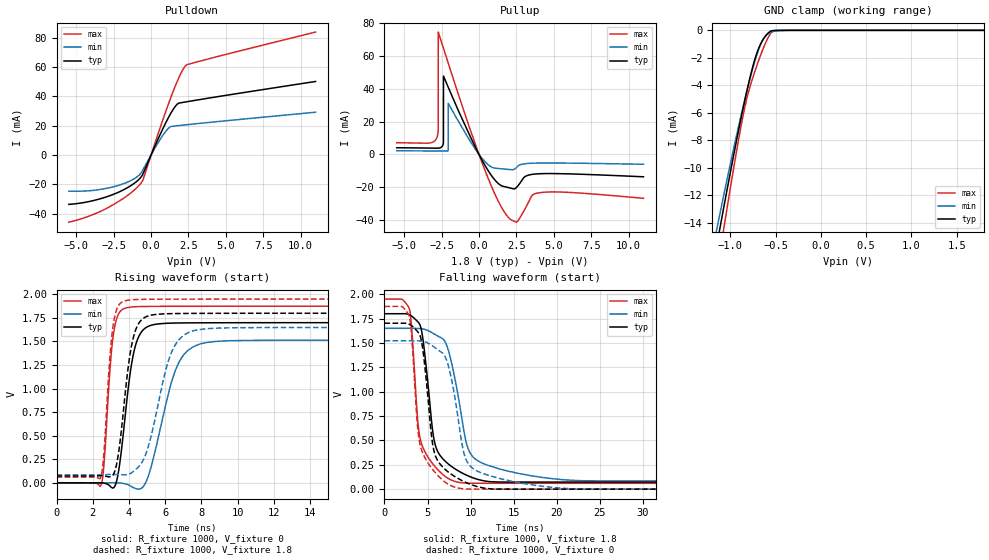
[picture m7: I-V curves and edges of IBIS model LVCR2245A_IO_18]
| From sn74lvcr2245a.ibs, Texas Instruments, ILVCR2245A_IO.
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[Model]   LVCR2245A_IO_18
Model_type  I/O
Vinl=0.5775
Vinh=1.2675
Enable   Active-Low
Vref =   0
Rref =   1000
Cref =   30p
Vmeas =   0.9
| variable   typ   min   max
C_comp   5.81pF   5.64pF   6.29pF
| C_pullup   5.68pF   4.72pF   6.93pF
| C_pulldown   4.75pF   4.06pF   6.38pF
| C_tri-state   5.81pF   5.64pF   6.29pF
[Temperature Range]   40   100   -40
| Ambient temperature   25   85   -40
[Voltage range]   1.8   1.65   1.95
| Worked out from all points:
|   slope of the pulldown table from 0 to 0.27 V, typ, clamps not added: 42.5 ohm
|   slope of the pullup table from 0 to 0.27 V, typ, clamps not added: 58.8 ohm
|   GND clamp passes 1 mA (typ) near -0.67 V on its own axis
|   rising waveform, R_fixture 1000, V_fixture 0: 20-80 % time 659ps typ, 1.2ns min, 405ps max; typ from 0 V to 1.7 V
|   falling waveform, R_fixture 1000, V_fixture 1.8: 20-80 % time 1.44ns typ, 2.12ns min, 1.2ns max; typ from 1.8 V to 0.073 V
|   rising waveform, R_fixture 1000, V_fixture 1.8: 20-80 % time 647ps typ, 1.17ns min, 400ps max; typ from 0.073 V to 1.8 V
|   falling waveform, R_fixture 1000, V_fixture 0: 20-80 % time 1.37ns typ, 1.91ns min, 1.21ns max; typ from 1.7 V to 0 V
[GND Clamp]
| LVCR2245A_IO_18
|   Voltage   I(typ)   I(min)   I(max)
-5.5V     -191mA     -172.6mA   -219.2mA
-1.155V   -15.81mA   -14.6mA    -17.82mA
-1.115V   -14.36mA   -13.31mA   -16.15mA
-1.08V    -13.11mA   -12.19mA   -14.7mA
-1.045V   -11.88mA   -11.09mA   -13.26mA
-935mV    -8.103mA   -7.723mA   -8.901mA
-855mV    -5.522mA   -5.416mA   -6.041mA
-810mV    -4.171mA   -4.195mA   -4.729mA
-745mV    -2.448mA   -2.581mA   -3.287mA
-640mV    -679.9uA   -662.4uA   -1.354mA
-530mV    -22.6uA    -93.97uA   -52.84uA
1.8V      36.78pA    10.02nA    -1.384nA
[Pulldown]
| LVCR2245A_IO_18
|   Voltage   I(typ)   I(min)   I(max)
-5.5V     -33.74mA   -24.8mA    -45.91mA
-3.97V    -31.41mA   -24.29mA   -41.06mA
-2.605V   -27.23mA   -21.94mA   -34.38mA
-1.375V   -21.08mA   -17.61mA   -26.1mA
-670mV    -15.02mA   -12.24mA   -19.16mA
-520mV    -12.37mA   -9.63mA    -16.31mA
495mV     11.51mA    8.797mA    15.32mA
1.11V     24.56mA    17.67mA    33.39mA
1.745V    34.65mA    19.96mA    50.16mA
2.1V      35.85mA    20.36mA    57.82mA
2.355V    36.3mA     20.63mA    61.42mA
11V       50.2mA     29.22mA    83.93mA
[Pullup]
| LVCR2245A_IO_18
|   Voltage   I(typ)   I(min)   I(max)
-5.5V     4.122mA    2.276mA    7.196mA
-2.81V    3.859mA    2.118mA    10.5mA
-2.73V    3.868mA    2.112mA    14.82mA
-2.725V   3.87mA     2.111mA    74.73mA
-2.385V   7.027mA    2.085mA    65.04mA
-2.38V    7.733mA    2.085mA    64.9mA
-2.375V   47.86mA    2.084mA    64.76mA
-2.06V    41.1mA     2.782mA    55.79mA
-2.055V   40.99mA    31.29mA    55.65mA
2.09V     -20.49mA   -9.224mA   -39.54mA
4.04V     -11.77mA   -5.224mA   -23.37mA
11V       -13.62mA   -5.978mA   -26.77mA
[Ramp]
| LVCR2245A_IO_18
| variable   typ   min   max
dV/dt_r   1.05/6.80E-10   0.95/1.24E-09   1.15/4.18E-10
dV/dt_f   1.04/1.44E-09   0.94/2.12E-09   1.13/1.20E-09
R_load = 1000
[Rising Waveform]
| LVCR2245A_IO_18
R_fixture =   1000
C_fixture =   0
L_fixture =   0
V_fixture =   0
V_fixture_min = 0
V_fixture_max = 0
|   Time   V(typ)   V(min)   V(max)
0s        702pV      3.493nV    28.21nV
2.46ns    -115.1uV   -529uV     -22.19mV
3.155ns   -51.34mV   393.3uV    1.591V
3.465ns   169.6mV    -1.365mV   1.805V
3.915ns   929.8mV    -16.65mV   1.859V
4.32ns    1.427V     -56.76mV   1.868V
4.83ns    1.631V     -29.83mV   1.871V
6.655ns   1.696V     1.235V     1.873V
8.27ns    1.698V     1.488V     1.874V
50ns      1.7V       1.515V     1.874V
[Falling Waveform]
| LVCR2245A_IO_18
R_fixture =   1000
C_fixture =   0
L_fixture =   0
V_fixture =   1.8
V_fixture_min = 1.65
V_fixture_max = 1.95
|   Time   V(typ)   V(min)   V(max)
0s        1.8V       1.65V      1.95V
2.905ns   1.788V     1.651V     1.845V
4.11ns    1.688V     1.648V     536.1mV
5.815ns   483.5mV    1.591V     237.4mV
7.025ns   289.2mV    1.515V     132.6mV
7.825ns   230.4mV    1.282V     90.83mV
9.715ns   136.2mV    416mV      61.21mV
12.21ns   77.04mV    238.6mV    60.45mV
22.18ns   72.71mV    88.93mV    60.22mV
50ns      72.58mV    84.7mV     60.16mV
[Rising Waveform]
| LVCR2245A_IO_18
R_fixture =   1000
C_fixture =   0
L_fixture =   0
V_fixture =   1.8
V_fixture_min = 1.65
V_fixture_max = 1.95
|   Time   V(typ)   V(min)   V(max)
0s        72.55mV    84.59mV    60.15mV
2.43ns    75.05mV    85.14mV    52.86mV
2.6ns     74mV       86.19mV    273.3mV
3.125ns   84.75mV    88.98mV    1.666V
3.44ns    337.2mV    88.19mV    1.885V
3.88ns    1.103V     85.29mV    1.936V
4.725ns   1.735V     220.2mV    1.947V
6.36ns    1.795V     1.389V     1.949V
7.82ns    1.798V     1.625V     1.949V
50ns      1.8V       1.65V      1.95V
[Falling Waveform]
| LVCR2245A_IO_18
R_fixture =   1000
C_fixture =   0
L_fixture =   0
V_fixture =   0
V_fixture_min = 0
V_fixture_max = 0
|   Time   V(typ)   V(min)   V(max)
0s        1.702V     1.522V     1.875V
2.905ns   1.691V     1.523V     1.767V
4.085ns   1.586V     1.521V     477.7mV
4.535ns   1.377V     1.516V     352.6mV
5.725ns   401.4mV    1.461V     187.8mV
7.035ns   203.4mV    1.361V     73.01mV
7.855ns   147.4mV    1.096V     30.39mV
9.465ns   68.65mV    305.2mV    2.014mV
12.37ns   2.528mV    133.4mV    305.2uV
50ns      28.83uV    105.2uV    10.64uV
